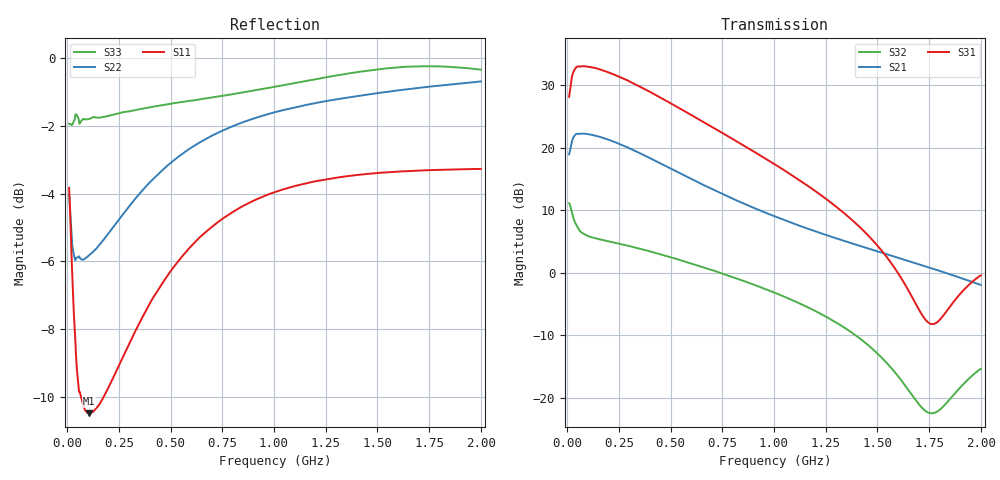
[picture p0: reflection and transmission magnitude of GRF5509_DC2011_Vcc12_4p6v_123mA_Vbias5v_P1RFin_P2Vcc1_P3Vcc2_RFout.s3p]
!Keysight Technologies,N5244B,MY57181157,A.18.40.03
!Date: Wednesday, April 29, 2026 14:25:29
!Correction: S11(C  3-Port  )
!S12(C  3-Port  )
!S13(C  3-Port  )
!S21(C  3-Port  )
!S22(C  3-Port  )
!S23(C  3-Port  )
!S31(C  3-Port  )
!S32(C  3-Port  )
!S33(C  3-Port  )
!S3P File: Measurements: <S11,S12,S13>,
!<S21,S22,S23>,
!<S31,S32,S33>:
# Hz S  dB  R 50
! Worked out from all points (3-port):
!   1991 points, 10 MHz to 2 GHz, reference 50 ohm
!   strongest paths, dB at 10 MHz, 507 MHz, 1.005 GHz, 1.503 GHz, 2 GHz:
!     S31: 28.2, 27.0, 17.4, 4.3, -0.4
!     S21: 19.0, 16.6, 9.0, 3.4, -1.9
!     S32: 11.2, 2.5, -3.2, -13.0, -15.4
!   lowest |S11| = -10.5 dB at 105 MHz (marker M1), VSWR 1.85, Z = 30.3 - j14.4 ohm
!   |S11| at or under -10 dB: 67.15 MHz to 177.3 MHz (110.2 MHz wide, 90.1 % of centre)
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1e7  -3.83 -54.4  -22.22 -34.5  -56.43 -96.4
     18.98 -137.1  -4.02 -79.0  -32.00 -82.2
     28.18 78.3  11.17 -173.4  -1.94 -112.4
3e7  -7.14 -91.7  -26.69 -42.6  -62.69 123.0
     21.64 -161.7  -5.72 -123.2  -42.92 146.4
     32.11 32.6  8.88 162.2  -1.90 -147.5
4.4e7  -8.85 -109.5  -28.77 -42.5  -64.51 156.0
       22.22 -172.8  -5.91 -137.2  -42.53 -37.1
       32.90 16.4  7.75 158.5  -1.66 -158.0
1.05e8  -10.49 -133.7  -32.36 -31.4  -70.44 62.8
        22.19 163.5  -5.83 -157.2  -50.97 29.2
        32.98 -16.7  5.86 154.5  -1.80 -169.4
1.73e8  -10.05 -139.0  -33.36 -26.1  -70.15 -121.7
        21.63 146.1  -5.39 -161.6  -45.51 44.1
        32.41 -39.0  5.26 147.7  -1.74 -172.1
2.54e8  -9.04 -140.6  -33.97 -24.8  -65.64 119.3
        20.63 129.1  -4.74 -163.8  -42.45 42.1
        31.37 -60.5  4.66 138.4  -1.62 -172.9
4.76e8  -6.51 -145.1  -35.17 -27.2  -60.69 83.6
        17.12 94.6  -3.22 -169.7  -39.72 32.2
        27.61 -106.7  2.76 113.3  -1.37 -173.1
6.68e8  -5.15 -150.7  -36.18 -28.8  -58.43 80.1
        13.94 74.9  -2.39 -174.9  -39.41 27.6
        23.98 -136.7  0.82 94.2  -1.19 -172.9
1.005e9  -3.95 -159.9  -37.57 -29.6  -54.90 86.5
         9.03 52.8  -1.59 178.0  -40.17 29.6
         17.36 -177.5  -3.18 65.5  -0.84 -173.3
2e9  -3.27 -178.7  -40.48 -43.3  -48.29 91.3
     -1.90 10.3  -0.68 156.3  -34.90 71.2
     -0.40 -126.5  -15.36 122.7  -0.34 172.2
